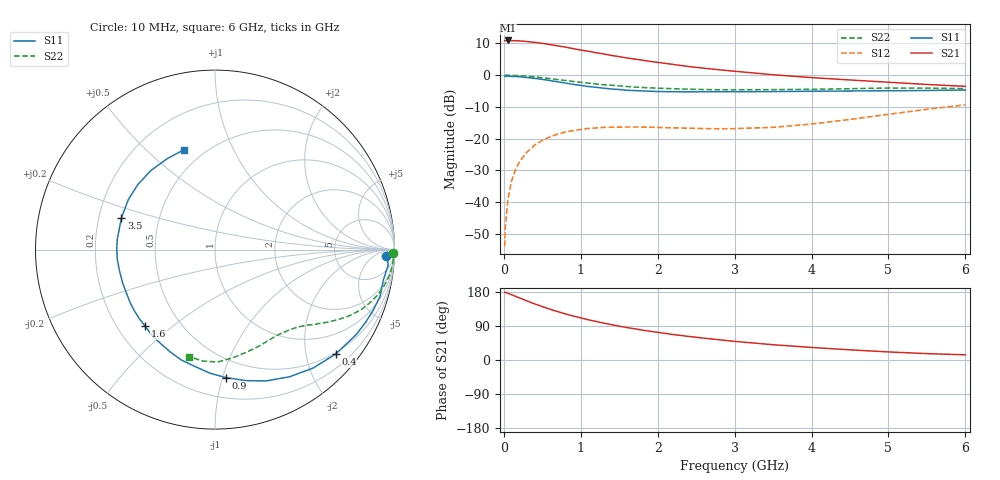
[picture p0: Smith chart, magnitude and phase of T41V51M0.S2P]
! Infineon Technologies  Discrete & RF Semiconductors
! BFR182T
! Si NPN RF Bipolar Junction Transistor in SC75
! VCE = 1.5 V  IC = 1 mA
! Common Emitter S-Parameters:  October  1999
# GHz  S  MA  R  50
!  f  S11  S21  S12  S22
! GHz  MAG  ANG  MAG  ANG  MAG  ANG  MAG  ANG
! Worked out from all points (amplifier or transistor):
!   36 points, 10 MHz to 6 GHz, reference 50 ohm
!   highest |S21| = 11.0 dB at 50 MHz (marker M1)
!   |S21| within 3 dB of that: start of sweep to 992.1 MHz
!   unconditionally stable (mu >= 1): 2.347 GHz to 4.67 GHz
!   at 250 MHz: K = 0.10, MSG = 18.3 dB, |S12| = -25.8 dB
!   at 1.4 GHz: K = 0.60, MSG = 11.3 dB, |S12| = -16.5 dB
!   at 6 GHz: K = 0.87, MSG = 2.9 dB, |S12| = -9.4 dB
!   S11 on the Smith chart (normalised r, x): 10 MHz: 26, -20; 400 MHz: 0.47, -2.62; 900 MHz: 0.35, -1.02; 1.6 GHz: 0.32, -0.40; 3.5 GHz: 0.30, +0.15; 6 GHz: 0.39, +0.66
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0.01  0.9529 -2.1  3.499 178.7  0.002 81.8  0.9925 -1.2
0.02  0.9596 -0.8  3.488 178.9  0.004 92.2  0.9999 -0.9
0.05  0.9683 -5.3  3.528 176.0  0.0105 91.5  0.997 -2.1
0.1  0.9534 -10.1  3.496 172.4  0.0214 86.8  0.9932 -4.2
0.15  0.9555 -15.9  3.5 168.1  0.032 80.6  0.9886 -6.3
0.25  0.9318 -25.8  3.435 160.1  0.051 74.4  0.9731 -10.3
0.4  0.8896 -40.8  3.296 148.2  0.0787 66.3  0.9387 -15.9
0.5  0.8572 -50.3  3.173 141.0  0.0933 60.8  0.911 -19.1
0.6  0.8214 -59.6  3.039 134.0  0.1065 56.2  0.8821 -22.1
0.7  0.7852 -68.7  2.901 127.7  0.1174 52.2  0.8521 -24.7
0.8  0.75 -76.8  2.773 121.7  0.1264 47.9  0.8234 -27.1
0.9  0.7153 -85.2  2.625 116.1  0.1331 44.6  0.7954 -29.1
1.1  0.6602 -99.9  2.38 105.9  0.1442 38.9  0.7482 -32.6
1.4  0.6049 -120.0  2.045 93.2  0.1504 32.7  0.6924 -37.1
1.6  0.5771 -132.4  1.868 85.6  0.1523 30.0  0.662 -39.5
1.8  0.5638 -143.0  1.726 78.8  0.1516 28.6  0.6386 -42.2
2.2  0.5471 -160.1  1.477 67.3  0.1474 28.2  0.611 -46.9
2.8  0.5471 179.8  1.216 53.4  0.1426 32.5  0.5882 -55.4
3.5  0.5505 161.2  1.015 40.3  0.1501 43.3  0.591 -65.3
4.5  0.5625 139.9  0.839 26.8  0.2002 55.8  0.6112 -80.7
5.5  0.5724 117.7  0.713 16.8  0.289 57.4  0.6247 -96.3
6  0.5832 107.1  0.666 13.7  0.34 54.8  0.6134 -103.6
